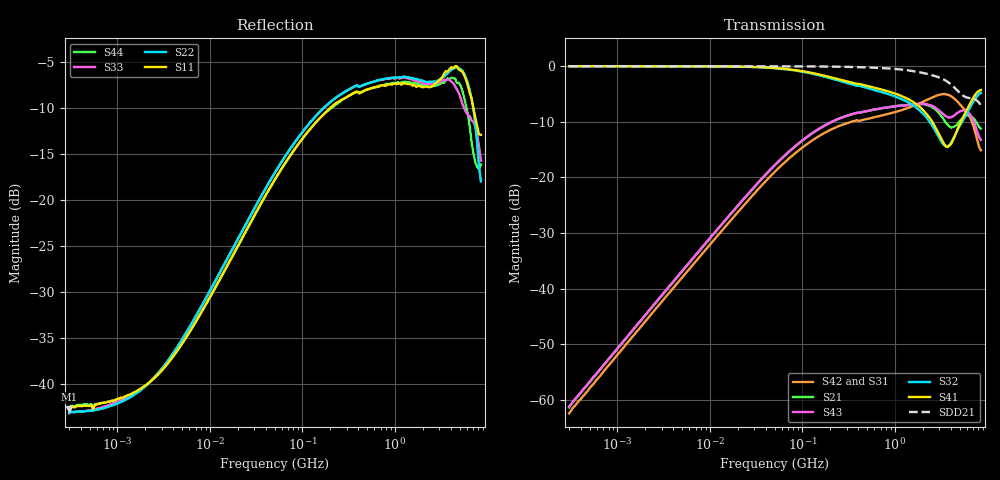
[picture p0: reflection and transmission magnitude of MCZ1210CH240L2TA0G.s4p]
! S-Parameter Data Generated by TDK Corporation
! Copyright(C) 2025 TDK Corporation.
! All Rights Reserved.
! TDK P/N: MCZ1210CH240L2TA0G (Signal Line Common Mode Choke/Filter)
! Property: |Zc|=24ohm at 100MHz
! Size(LxWxT): 1.25x1x0.5mm
! Model Type: s2p (Touchstone File Format Version 1.0)
! Frequency: DC=Yes Start=0.3MHz Stop=8500MHz 225points Log-sweep
! Model Generated on Feb. 6, 2025
! Terms and conditions regarding TDK Simulation Models:
! 1)This simulation model is being provided solely for informational
!  purposes. Please refer to the specifications of the products in
!  terms of detailed characteristics of such products.
! 2)In no event shall TDK Corporation of any of its subsidiaries be
!  liable for any loss or damage arising, directly or indirectly,
!  from any information contained in this simulation model, including,
!  but not limited to loss or damages arising from any inaccuracies,
!  omissions or errors in connection with such information.
! 3)Any and all copyrights on this simulation model are owned by
!  TDK Corporation.  Duplication or redistribution of this simulation
!  model without prior written permission from TDK Corporation
!  is prohibited.
! 4)This simulation model is subject to any modification or change
!  without any prior notice.
! 5)Neither TDK Corporation nor any of its subsidiaries shall make any
!  warranty, express or implied, including but not limited to the
!  correctness, implied warranties of merchantability and fitness for
!  a particular purpose with respect to this simulation models.
! 6)The use of this simulation model shall be deemed to have consented
!  to the terms and conditions hereof.
! Port Assignments:
!  1 ---@@@--- 4
!  2 ---@@@--- 3
! Applicable Conditions:
!  Temperature = 25 degC
!  DC Bias Current = 0 A
!  Small Signal Operation
# Hz S MA R 50
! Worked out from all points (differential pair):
!   224 points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, 300 kHz to 8.5 GHz, reference 50 ohm
!   strongest paths, dB at 300 kHz, 3.937 MHz, 51.67 MHz, 678.1 MHz, 8.5 GHz:
!     S41: -0.1, -0.1, -0.4, -4.1, -4.3
!     S32: -0.1, -0.1, -0.4, -4.6, -4.8
!     S43: -61.2, -38.9, -17.6, -7.7, -13.3
!     S21: -61.3, -38.9, -17.6, -7.7, -11.3
!     S42: -62.4, -40.0, -18.8, -9.0, -15.1
!     S31: -62.3, -40.1, -18.9, -8.8, -15.8
!   taken as a pair (ports 1,2 in; 4,3 out), SDD21 dB: -0.1, -0.1, -0.1, -0.4, -7.1
!   lowest |S11| = -42.7 dB at 300 kHz (marker M1), VSWR 1.01, Z = 50.7 + j0.0459 ohm
!   |S11| at or under -10 dB: start of sweep to 197.9 MHz; 7.05 GHz to end of sweep
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300000  0.007333 3.5  0.0008772 90.2  0.000783 -90.9  0.9923 -0.1
        0.0008602 89.1  0.007019 7.3  0.9933 -0.1  0.0007688 -89.9
        0.0007654 -90.1  0.9916 -0.0  0.006973 8.5  0.0008874 90.3
        0.993 -0.1  0.0007626 -89.5  0.000876 89.9  0.007364 5.7
3128670  0.01216 47.5  0.00906 87.8  0.007942 -92.5  0.9912 -0.6
         0.009028 88.0  0.01242 52.2  0.9924 -0.6  0.0079 -92.3
         0.007897 -92.4  0.9915 -0.6  0.01247 51.9  0.009015 87.9
         0.9924 -0.6  0.007944 -92.4  0.009079 87.8  0.01215 47.5
1.420669e8  0.2676 45.7  0.2644 45.9  0.2285 -142.3  0.8459 -16.8
            0.2631 46.2  0.2894 45.3  0.835 -18.2  0.226 -142.3
            0.2275 -142.3  0.8339 -18.4  0.2898 45.3  0.2626 46.0
            0.8467 -16.8  0.2271 -142.5  0.2638 46.0  0.2675 45.5
1.02567e9  0.4297 2.6  0.4375 7.6  0.4013 134.0  0.56 -42.5
           0.4354 8.0  0.4644 0.2  0.5282 -45.6  0.3842 134.1
           0.3994 134.2  0.5277 -45.8  0.4608 -1.7  0.4304 8.1
           0.5605 -42.4  0.3863 133.8  0.4331 8.1  0.4332 0.9
3.548748e9  0.5024 -32.6  0.3111 -19.2  0.5625 30.9  0.1896 -168.0
            0.3098 -18.4  0.4782 -41.1  0.1904 -176.6  0.5541 30.2
            0.5597 31.2  0.1904 -177.2  0.45 -42.9  0.3528 -14.2
            0.1896 -167.6  0.5562 29.7  0.3543 -14.1  0.4478 -37.3
6.161135e9  0.4173 -74.9  0.3615 -8.5  0.3616 -23.2  0.4199 60.0
            0.3614 -7.3  0.4304 -82.3  0.3926 56.1  0.3665 -28.3
            0.3611 -23.4  0.3906 54.8  0.2898 -83.2  0.3805 -24.1
            0.4228 60.8  0.3689 -28.8  0.3838 -23.2  0.2929 -91.4
8.5e9  0.2267 -111.3  0.2742 -14.0  0.163 -14.4  0.605 6.3
       0.2736 -13.8  0.1267 -101.7  0.5744 0.8  0.1735 -26.1
       0.1618 -14.6  0.5722 0.5  0.1642 -83.2  0.214 -21.6
       0.6069 6.4  0.1749 -26.1  0.2163 -21.2  0.1566 -92.2
